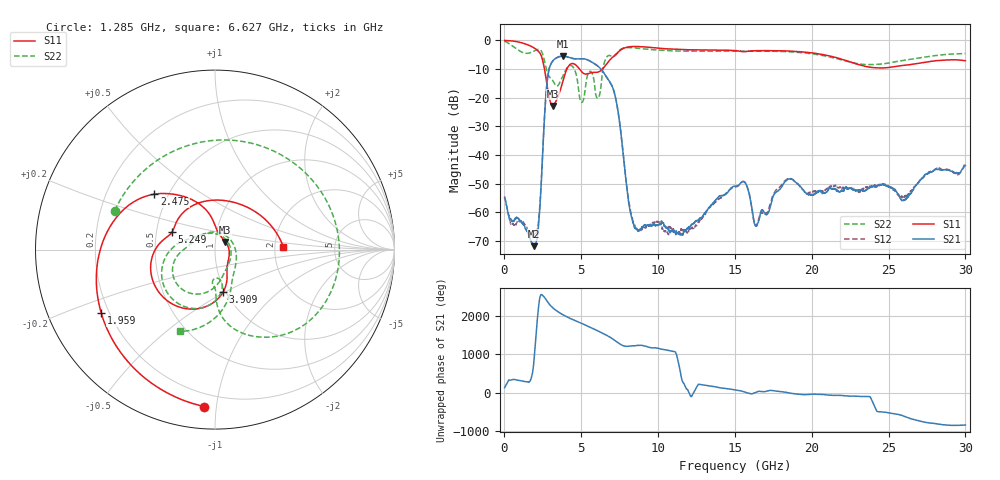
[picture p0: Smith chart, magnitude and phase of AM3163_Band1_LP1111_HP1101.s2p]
!Agilent Technologies,E8364B,MY43040894,A.07.50.67
!Agilent E8364B: A.07.50.67
!Date: Thursday, August 20, 2020 11:59:42
!Correction: S11(Full 2 Port(1,2))
!S21(Full 2 Port(1,2))
!S12(Full 2 Port(1,2))
!S22(Full 2 Port(1,2))
!S2P File: Measurements: S11, S21, S12, S22:
# Hz S  dB  R 50
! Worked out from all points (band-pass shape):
!   3201 points, 10 MHz to 30 GHz, reference 50 ohm
!   highest |S21| = -5.54 dB at 3.806 GHz (marker M1); lowest = -71.8 dB at 1.922 GHz (marker M2)
!   |S21| within 3 dB of the highest: 2.999 GHz to 5.963 GHz (2.964 GHz wide, 66.1 % of centre)
!   lowest |S11| = -22.9 dB at 3.131 GHz (marker M3), VSWR 1.15, Z = 55.9 + j4.85 ohm
!   |S11| at or under -10 dB: 2.605 GHz to 4.068 GHz (1.463 GHz wide, 43.8 % of centre); 4.877 GHz to 6.388 GHz (1.511 GHz wide, 26.8 % of centre)
!   |S22| runs from -21.7 to -0.3 dB; largest |S21 - S12| = 0.0057
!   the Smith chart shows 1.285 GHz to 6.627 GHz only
!   S11 on the Smith chart (normalised r, x): 1.285 GHz: 0.12, -0.93; 1.959 GHz: 0.17, -0.25; 2.475 GHz: 0.42, +0.33; 3.909 GHz: 0.97, -0.49; 5.249 GHz: 0.60, +0.13; 6.627 GHz: 2.22, +0.09
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1e7  -0.08 -5.0  -55.06 125.6  -54.32 -157.9  -0.33 -11.6
5.723125e8  -0.29 -41.1  -62.91 -21.8  -64.16 -21.2  -2.14 -91.6
1.284575e9  -1.14 -93.8  -64.58 -69.4  -64.00 -74.8  -4.44 158.8
1.921862e9  -2.66 -147.3  -71.79 114.2  -67.68 -39.7  -3.78 51.9
1.95935e9  -2.79 -151.0  -71.23 -57.0  -67.31 37.8  -3.68 45.3
2.474803e9  -6.78 137.6  -40.88 24.2  -40.49 25.5  -4.68 -56.3
3.130834e9  -22.88 37.0  -7.32 59.1  -7.34 59.0  -13.96 -92.8
3.805609e9  -14.25 -70.5  -5.54 -127.6  -5.57 -127.5  -12.30 -82.3
3.9087e9  -12.33 -79.4  -5.58 -150.3  -5.61 -150.2  -11.16 -87.9
5.014581e9  -10.91 167.3  -6.43 8.4  -6.41 8.3  -21.62 53.9
5.248878e9  -11.77 157.7  -6.55 -34.2  -6.56 -34.3  -17.30 -66.8
5.951769e9  -11.20 95.5  -8.50 -164.0  -8.51 -164.1  -19.14 135.6
6.626544e9  -8.39 2.5  -12.64 59.5  -12.74 59.7  -6.12 -112.9
7.526244e9  -3.54 -102.4  -29.96 -176.5  -29.98 -175.4  -3.32 -171.0
8.379084e9  -2.18 -171.9  -63.63 142.0  -63.23 146.6  -2.65 136.1
1.000979e10  -2.77 100.6  -64.53 74.6  -63.21 70.6  -3.45 65.5
1.227778e10  -3.36 9.7  -64.06 -33.0  -65.53 -119.6  -3.84 -15.1
1.5005e10  -3.59 -74.1  -50.88 67.1  -51.18 68.6  -3.79 -92.5
1.638267e10  -3.64 -104.9  -64.68 8.6  -64.53 11.5  -3.80 -126.1
2.000958e10  -4.40 162.6  -53.93 -45.8  -52.60 -54.7  -4.71 135.5
2.500479e10  -9.50 -63.1  -50.97 -171.3  -51.07 -168.9  -7.96 -93.2
3e10  -7.15 103.7  -43.68 -130.4  -42.84 -130.7  -4.64 100.1
